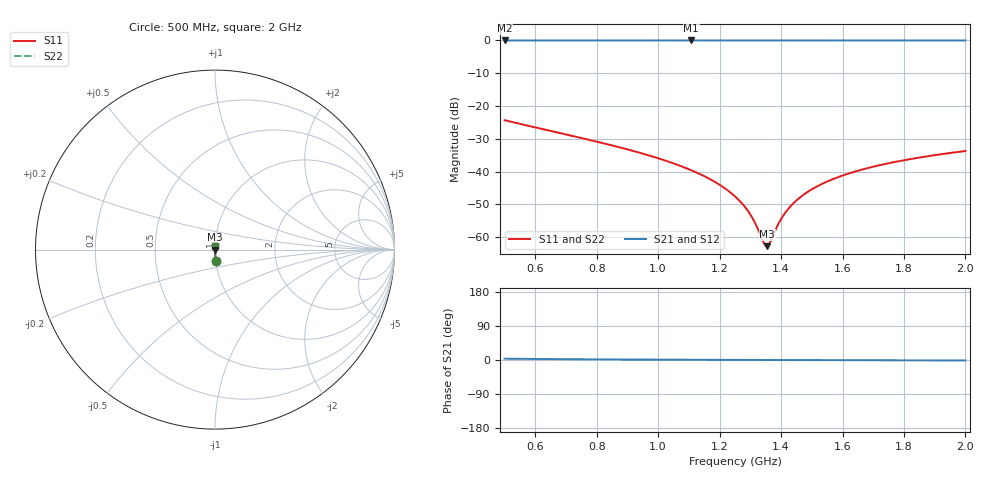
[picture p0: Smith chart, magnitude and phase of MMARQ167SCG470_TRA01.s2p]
! MMARQ167SCG470_TRA01  S-PARAMETER MODEL  ( General Type )
! Model Generated by TAIYO YUDEN Corporation (http://www.ty-top.com)
! Version 1.0
! TAIYO YUDEN Control No. 150305
! Copyright(c) 2015 TAIYO YUDEN CO.,LTD. All Rights Reserved.
! Product Description (link to TY-COMPAS)
! https://ds.yuden.co.jp/TYCOMPAS/or/detail?pn=MMARQ167SCG470JTRA01&u=M
! Products Name : Multilayer Ceramic Capacitors
! Characteristics :
!  Capacitance : 47 pF , Rated Voltage : 250V , TCC : CG / C0G
!  Case Size : 1.6 x 0.8 / 0.063 x 0.031 [mm/inch] , Thickness : 0.7 / 0.028 [mm/inch]
!  (Conditions: Temperature = 25 degC , DC Bias Current/Voltage = 0A / 0V)
! External Node Assignments :
!  1  o---| |---o  2
! GND o---------o GND
! Frequency Range : 500MHz  -  2GHz  [ 401 STEP ]
# MHz S RI R 50
! Freq[MHz].  S11 Real  S11 Imag  S21 Real  S21 Imag  S12 Real  S12 Imag  S22 Real  S22 Imag
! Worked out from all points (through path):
!   401 points, 500 MHz to 2 GHz, reference 50 ohm
!   highest |S21| = -0.01 dB at 1.107 GHz (marker M1); lowest = 0.0 dB at 500 MHz (marker M2)
!   lowest |S11| = -62.7 dB at 1.355 GHz (marker M3), VSWR 1.00, Z = 50.1 + j0.00471 ohm
!   |S11| at or under -10 dB: start of sweep to end of sweep
!   |S22| runs from -62.7 to -24.3 dB; largest |S21 - S12| = 0
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500  0.00401 -0.0607  0.996 0.0607  0.996 0.0607  0.00401 -0.0607
751.25  0.00148 -0.0324  0.9985 0.0324  0.9985 0.0324  0.00148 -0.0324
1002.5  0.000805 -0.0158  0.9992 0.0158  0.9992 0.0158  0.000805 -0.0158
1107.5  0.000717 -0.0105  0.9993 0.0105  0.9993 0.0105  0.000717 -0.0105
1190  0.000694 -0.0067  0.9993 0.0067  0.9993 0.0067  0.000694 -0.0067
1250  0.000695 -0.00413  0.9993 0.00413  0.9993 0.00413  0.000695 -0.00413
1272.5  0.000699 -0.00321  0.9993 0.00321  0.9993 0.00321  0.000699 -0.00321
1295  0.000705 -0.0023  0.9993 0.0023  0.9993 0.0023  0.000705 -0.0023
1317.5  0.000713 -0.0014  0.9993 0.0014  0.9993 0.0014  0.000713 -0.0014
1343.75  0.000723 -0.000384  0.9993 0.000384  0.9993 0.000384  0.000723 -0.000384
1351.25  0.000727 -9.62e-05  0.9993 9.62e-05  0.9993 9.62e-05  0.000727 -9.62e-05
1355  0.000729 4.71e-05  0.9993 -4.71e-05  0.9993 -4.71e-05  0.000729 4.71e-05
1366.25  0.000734 0.000475  0.9993 -0.000475  0.9993 -0.000475  0.000734 0.000475
1396.25  0.00075 0.0016  0.9992 -0.0016  0.9992 -0.0016  0.00075 0.0016
1422.5  0.000766 0.00256  0.9992 -0.00256  0.9992 -0.00256  0.000766 0.00256
1456.25  0.00079 0.00377  0.9992 -0.00377  0.9992 -0.00377  0.00079 0.00377
1501.25  0.000824 0.00535  0.9992 -0.00535  0.9992 -0.00535  0.000824 0.00535
1550  0.000866 0.00701  0.9991 -0.00701  0.9991 -0.00701  0.000866 0.00701
1606.25  0.00092 0.00886  0.9991 -0.00886  0.9991 -0.00886  0.00092 0.00886
1752.5  0.00108 0.0134  0.9989 -0.0134  0.9989 -0.0134  0.00108 0.0134
1868.75  0.00123 0.0169  0.9988 -0.0169  0.9988 -0.0169  0.00123 0.0169
2000  0.00142 0.0206  0.9986 -0.0206  0.9986 -0.0206  0.00142 0.0206
